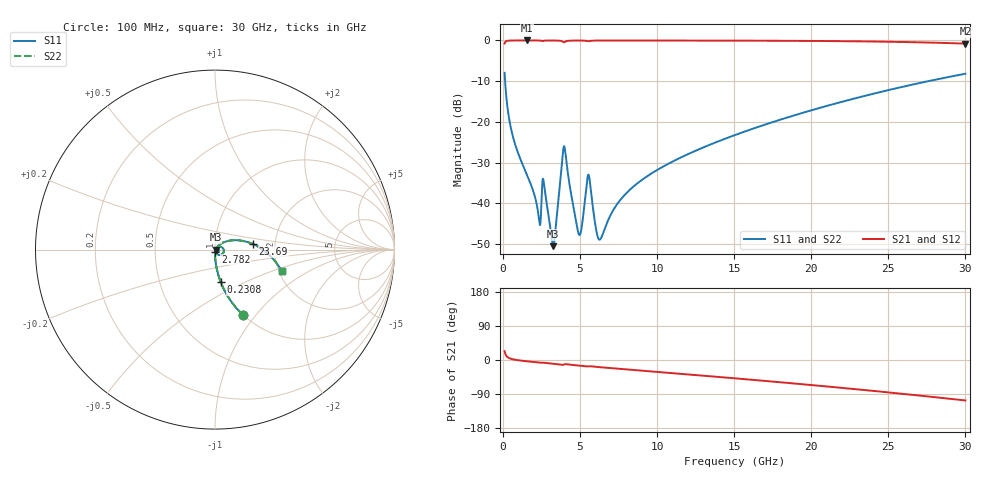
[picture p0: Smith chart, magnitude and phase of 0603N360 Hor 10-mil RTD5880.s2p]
# GHz S MA R 50
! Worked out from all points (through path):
!   3201 points, 100 MHz to 30 GHz, reference 50 ohm
!   highest |S21| = -0.01 dB at 1.558 GHz (marker M1); lowest = -0.8 dB at 30 GHz (marker M2)
!   group delay of S21, straight-line fit = 9.94 ps
!   lowest |S11| = -50.5 dB at 3.258 GHz (marker M3), VSWR 1.01, Z = 50.3 - j0.077 ohm
!   |S11| at or under -10 dB: 130.8 MHz to 27.6 GHz (27.47 GHz wide, 198 % of centre)
!   |S22| runs from -50.5 to -8.0 dB; largest |S21 - S12| = 0
!   S11 on the Smith chart (normalised r, x): 100 MHz: 1.00, -0.87; 230.8 MHz: 1.00, -0.38; 2.782 GHz: 1.01, -0.02; 23.69 GHz: 1.53, +0.10; 30 GHz: 2.07, -0.58
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0.1  0.3997 -66.7  0.9163 23.3  0.9163 23.3  0.3997 -66.7
0.2308125  0.185 -79.9  0.9823 10.0  0.9823 10.0  0.185 -79.9
0.660625  0.06369 -87.7  0.9972 1.7  0.9972 1.7  0.06369 -87.7
1.557625  0.02222 -90.5  0.9986 -3.4  0.9986 -3.4  0.02222 -90.5
2.323812  0.006535 -71.3  0.9971 -6.7  0.9971 -6.7  0.006535 -71.3
2.622813  0.01911 -55.1  0.9871 -7.1  0.9871 -7.1  0.01911 -55.1
2.781656  0.01145 -76.1  0.9957 -7.8  0.9957 -7.8  0.01145 -76.1
3.258188  0.002977 -14.9  0.997 -9.8  0.997 -9.8  0.002977 -14.9
3.8375  0.03404 28.5  0.9742 -12.9  0.9742 -12.9  0.03404 28.5
3.968313  0.05013 -18.3  0.9501 -11.7  0.9501 -11.7  0.05013 -18.3
4.818594  0.004938 -50.6  0.9959 -14.4  0.9959 -14.4  0.004938 -50.6
5.089563  0.004922 8.5  0.9954 -15.5  0.9954 -15.5  0.004922 8.5
5.528719  0.02247 -12.1  0.9775 -16.8  0.9775 -16.8  0.02247 -12.1
6.051969  0.004596 -41.6  0.9957 -18.1  0.9957 -18.1  0.004596 -41.6
6.285563  0.003587 -3.0  0.9965 -19.0  0.9965 -19.0  0.003587 -3.0
7.696469  0.01152 51.9  0.997 -23.8  0.997 -23.8  0.01152 51.9
10.06978  0.02612 51.6  0.9964 -31.6  0.9964 -31.6  0.02612 51.6
15.05  0.06891 38.4  0.9936 -48.4  0.9936 -48.4  0.06891 38.4
20.03956  0.1393 21.8  0.9852 -66.2  0.9852 -66.2  0.1393 21.8
23.69297  0.2136 8.3  0.9711 -80.2  0.9711 -80.2  0.2136 8.3
25.01978  0.2458 3.1  0.9631 -85.5  0.9631 -85.5  0.2458 3.1
30  0.3898 -17.8  0.9135 -106.7  0.9135 -106.7  0.3898 -17.8
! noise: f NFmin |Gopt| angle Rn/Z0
0.1  0.0002916  0.9183  0.3936  0.0007883
3.417  0.005226  0.8501  10.32  0.007364
6.743  0.006634  0.7775  20.28  0.005916
10.06  0.008198  0.7399  30.01  0.005899
13.39  0.01014  0.7263  39.54  0.006543
16.7  0.01213  0.72  48.77  0.007155
20.03  0.0142  0.7185  57.71  0.007716
23.35  0.01638  0.7205  66.3  0.008227
26.67  0.01873  0.7254  74.6  0.008699
30  0.02129  0.7327  82.58  0.009138
